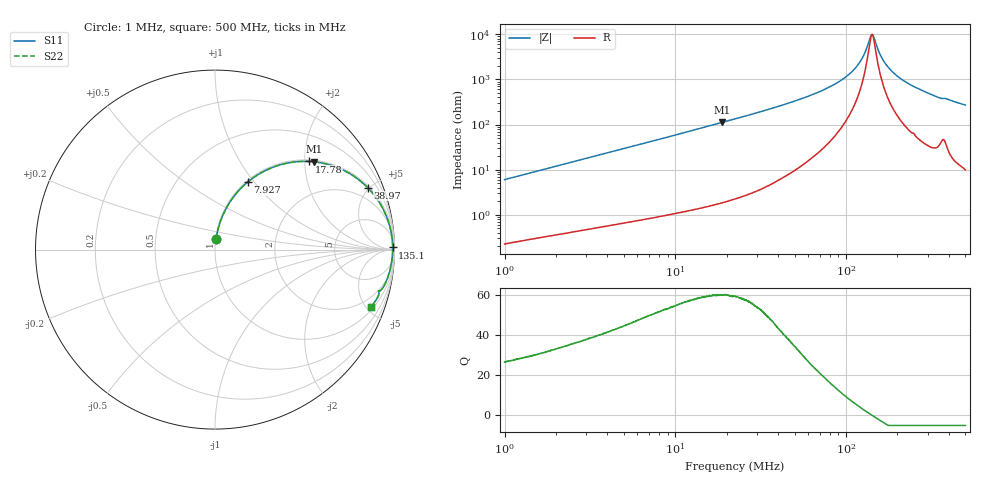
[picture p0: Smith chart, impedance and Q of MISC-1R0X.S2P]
!s-Parameter Generated by FASTRON Sdn. Bhd.
!FASTRON P/N : MISC-1R0X
!Keysight Technologies,E4991B,MY54100416,A.01.15
!Date: Mon Mar 16 10:24:53 2026
!Version  : Rev00 Mon Mar 16 10:24:53 2026
!Data & Calibration Information:
!PortZ  Port1:50+j0  Port2:50+j0
!When reading, reference impedance value at option line is always used.
! Remarks : This data is being provided solely for informational purposes.
!Freq	S11	S21	S12	S22
# Hz S dB R 50
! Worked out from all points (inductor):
!   1601 points, 1 MHz to 500 MHz, reference 50 ohm
!   read as one part in series: L = 954 nH near 1.032 MHz
!   highest Q = 60.3 at 18.85 MHz (marker M1), where L = 940 nH
!   self-resonance near 142.1 MHz
!   S11 on the Smith chart (normalised r, x): 1 MHz: 1.00, +0.12; 7.927 MHz: 1.02, +0.93; 17.78 MHz: 1.03, +2.10; 38.97 MHz: 1.11, +4.89; 135.1 MHz: open; 500 MHz: 1.20, -5.41
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1000000  -24.43 84.4  -0.04 -3.4  -0.04 -3.4  -24.43 84.4
2820919  -15.71 79.0  -0.16 -9.4  -0.16 -9.4  -15.71 79.0
5012396  -11.04 72.4  -0.41 -16.3  -0.41 -16.3  -11.04 72.4
7926736  -7.58 64.2  -0.91 -24.7  -0.91 -24.7  -7.58 64.2
7957584  -7.55 64.1  -0.92 -24.8  -0.92 -24.8  -7.55 64.1
1.778118e7  -2.88 43.2  -3.29 -45.8  -3.29 -45.8  -2.88 43.2
1.884792e7  -2.64 41.5  -3.57 -47.5  -3.57 -47.5  -2.64 41.5
2.236068e7  -2.02 36.6  -4.49 -52.4  -4.49 -52.4  -2.02 36.6
3.896776e7  -0.74 22.1  -8.50 -66.7  -8.50 -66.7  -0.74 22.1
6.307767e7  -0.28 12.2  -13.46 -75.4  -13.46 -75.4  -0.28 12.2
8.539853e7  -0.15 7.3  -17.95 -78.8  -17.95 -78.8  -0.15 7.3
1.057371e8  -0.10 4.1  -22.83 -78.5  -22.83 -78.5  -0.10 4.1
1.220791e8  -0.09 2.1  -28.48 -73.3  -28.48 -73.3  -0.09 2.1
1.350515e8  -0.09 0.7  -36.09 -50.9  -36.09 -50.9  -0.09 0.7
1.39856e8  -0.09 0.2  -39.50 -21.4  -39.50 -21.4  -0.09 0.2
1.437107e8  -0.09 -0.1  -39.78 14.6  -39.78 14.6  -0.09 -0.1
1.602216e8  -0.09 -1.6  -30.36 68.6  -30.36 68.6  -0.09 -1.6
1.77937e8  -0.11 -3.1  -25.20 75.8  -25.20 75.8  -0.11 -3.1
2.110998e8  -0.14 -5.5  -20.25 77.9  -20.25 77.9  -0.14 -5.5
2.685796e8  -0.22 -9.2  -15.90 76.4  -15.90 76.4  -0.22 -9.2
3.470608e8  -0.43 -13.7  -12.46 71.6  -12.46 71.6  -0.43 -13.7
5e8  -0.66 -20.0  -9.31 67.9  -9.31 67.9  -0.66 -20.0
